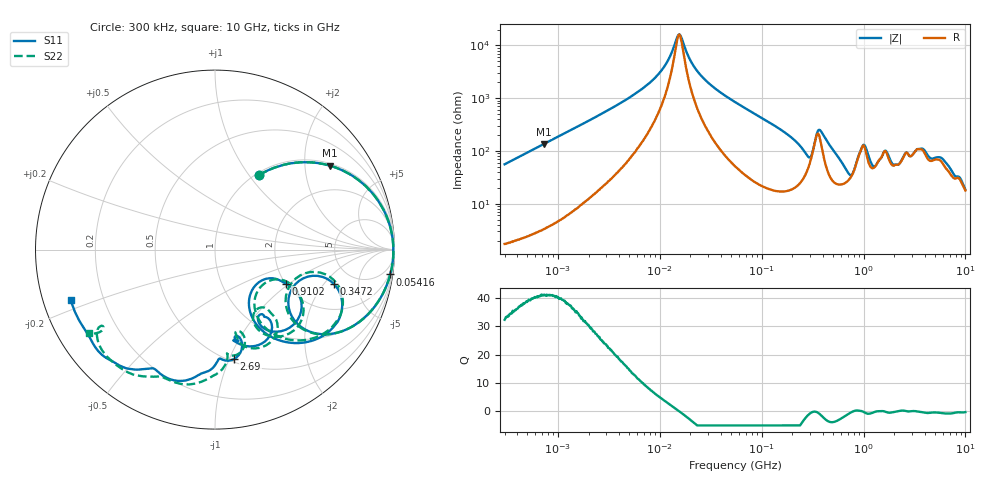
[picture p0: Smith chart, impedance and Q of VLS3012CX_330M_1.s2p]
! S-Parameter Data Generated by TDK Corporation
! Copyright(C) 2020 TDK Corporation.
! All Rights Reserved.
! TDK P/N: VLS3012CX-330M-1 (Inductor)
! Property: L=33uH at 1MHz
! Size(LxWxT): 3x3x1.2mm
! Model Type: s2p (Touchstone File Format Version 1.0)
! Frequency: DC=Yes Start=0.3MHz Stop=10000MHz 802points Log-sweep
! Model Generated on Aug. 18, 2020
! Port Assignments:
!  1 ---@@@--- 2
! Applicable Conditions:
!  Temperature = 25 degC
!  DC Bias Current = 0 A
!  Small Signal Operation
! Terms and conditions regarding TDK Simulation Models
! (1)This simulation model is being provided solely for informational purposes. Please refer to the specifications of the products in terms of detailed characteristics of such products.
! (2)In no event shall TDK Corporation of any of its subsidiaries be liable for any loss or damage arising, directly or indirectly,
!  From any information contained in this simulation model, including, but not limited to loss or damages arising from any inaccuracies, omissions or errors in connection with such information.
! (3)Any and all copyrights on this simulation model are owned by TDK Corporation.
!  Duplication or redistribution of this simulation model without prior written permission from TDK Corporation is prohibited.
! (4)This simulation model is subject to any modification or change without any prior notice.
! (5)Neither TDK Corporation nor any of its subsidiaries shall make any warranty, express or implied,
!  Including but not limited to the correctness, implied warranties of merchantability and fitness for a particular purpose with respect to this simulation models.
! (6)The use of this simulation model shall be deemed to have consented to the terms and conditions hereof.
# Hz S MA R 50
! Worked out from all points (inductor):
!   801 points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, 300 kHz to 10 GHz, reference 50 ohm
!   read as one part in series: L = 29.6 uH near 318.3 kHz
!   highest Q = 41 at 724.6 kHz (marker M1), where L = 29.5 uH
!   self-resonance near 15.36 MHz
!   S11 on the Smith chart (normalised r, x): 300 kHz: 1.03, +1.12; 54.16 MHz: 1, -14; 347.2 MHz: 3.48, -2.58; 910.2 MHz: 2.01, -0.94; 2.69 GHz: 0.53, -1.04; 10 GHz: 0.08, -0.17
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300000  0.4818 59.5  0.8617 -28.8  0.8614 -28.7  0.4812 59.5
724593  0.7931 36.1  0.5897 -52.5  0.5897 -52.5  0.7931 36.1
1713600  0.9458 17.2  0.2968 -71.1  0.2967 -71.0  0.9459 17.2
9671944  0.9929 1.7  0.03499 -77.7  0.03499 -77.7  0.9929 1.7
1.558358e7  0.9938 -0.5  0.006152 2.2  0.006139 2.4  0.9938 -0.5
2.441527e7  0.9934 -2.6  0.03388 77.3  0.03388 77.3  0.9934 -2.6
5.416364e7  0.9863 -8.1  0.1148 78.4  0.1148 78.4  0.9864 -8.1
5.477226e7  0.9861 -8.2  0.1163 78.4  0.1163 78.4  0.9861 -8.2
1.30774e8  0.9375 -20.9  0.2987 65.8  0.2987 65.8  0.9374 -20.9
2.195581e8  0.791 -36.5  0.5139 45.5  0.5138 45.5  0.7889 -36.7
3.126428e8  0.4986 -20.6  0.5302 2.0  0.5302 2.0  0.4784 -19.6
3.471693e8  0.6923 -16.2  0.3243 2.6  0.3243 2.6  0.6804 -14.2
5.046115e8  0.6832 -49.7  0.5871 28.2  0.587 28.2  0.685 -47.7
7.152593e8  0.3679 -59.0  0.735 -1.3  0.735 -1.3  0.3836 -55.0
9.101824e8  0.4381 -25.7  0.5203 -23.4  0.5203 -23.4  0.5046 -26.4
1.085776e9  0.5952 -48.7  0.4922 -2.1  0.4923 -2.1  0.6022 -53.7
1.387199e9  0.4514 -53.5  0.5758 -26.6  0.5757 -26.6  0.4258 -49.4
1.767019e9  0.577 -69.1  0.4846 -22.3  0.4848 -22.3  0.5947 -67.7
2.69003e9  0.6194 -80.2  0.4047 -50.8  0.4047 -50.8  0.5987 -78.5
3.816223e9  0.7303 -100.2  0.2839 -57.2  0.2836 -57.2  0.7539 -98.2
5.930102e9  0.8215 -126.1  0.2431 -67.3  0.2432 -67.2  0.8289 -122.5
1e10  0.8509 -160.6  0.2233 -82.6  0.2232 -82.7  0.8445 -146.4
